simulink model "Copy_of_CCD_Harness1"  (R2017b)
settings: Solver=FixedStepDiscrete  StartTime=0.0  StopTime=10.0  FixedStep=0.01  RelTol=1e-3
undefined symbols (not defined in the file): sigbuilder_block

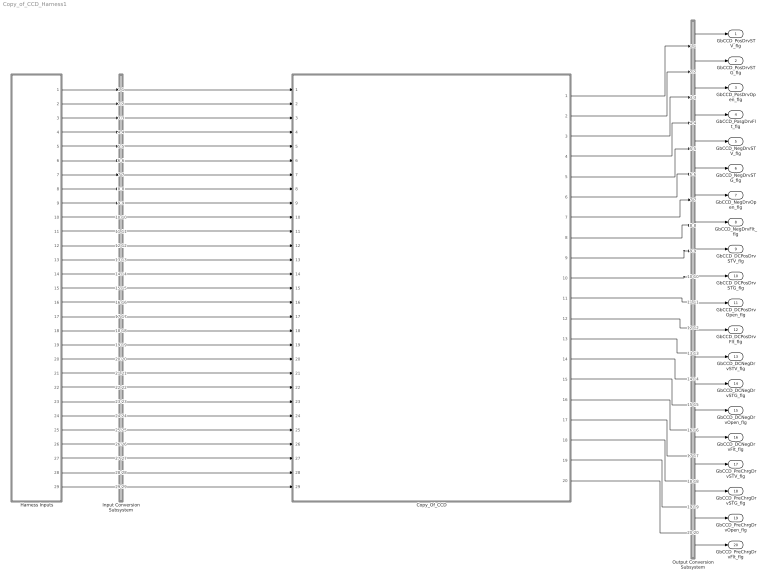
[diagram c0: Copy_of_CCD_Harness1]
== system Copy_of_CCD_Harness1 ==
  Copy_Of_CCD : ModelReference  ModelNameDialog=Copy_Of_CCD  SimulationMode=Normal  ModelReferenceVersion=1.11
  Harness Inputs : Subsystem  Tag=STV Subsys  LoadFcn=sigbuilder_block('load');  StartFcn=sigbuilder_block('start');  StopFcn=sigbuilder_block('stop');  ClipboardFcn=sigbuilder_block('clipboard');  mask(Sigbuilder block){tuvar=[0:10]}
      mask init:
      | if ~strcmp(get_param(bdroot(gcb),'SimulationStatus'),'stopped'),tuvar = sigbuilder_block('maskInit'); end
  Input Conversion Subsystem : Subsystem  Tag=__SLT_ICS__  Description=Signal spec. and routing
  Output Conversion Subsystem : Subsystem  Tag=__SLT_OCS__  Description=Signal spec. and routing
  GbCCD_PosDrvSTV_flg : Outport  OutDataTypeStr=boolean  PortDimensions=[1]
  GbCCD_PosDrvSTG_flg : Outport  Port=2  OutDataTypeStr=boolean  PortDimensions=[1]
  GbCCD_PosDrvOpen_flg : Outport  Port=3  OutDataTypeStr=boolean  PortDimensions=[1]
  GbCCD_PosgDrvFlt_flg : Outport  Port=4  OutDataTypeStr=boolean  PortDimensions=[1]
  GbCCD_NegDrvSTV_flg : Outport  Port=5  OutDataTypeStr=boolean  PortDimensions=[1]
  GbCCD_NegDrvSTG_flg : Outport  Port=6  OutDataTypeStr=boolean  PortDimensions=[1]
  GbCCD_NegDrvOpen_flg : Outport  Port=7  OutDataTypeStr=boolean  PortDimensions=[1]
  GbCCD_NegDrvFlt_flg : Outport  Port=8  OutDataTypeStr=boolean  PortDimensions=[1]
  GbCCD_DCPosDrvSTV_flg : Outport  Port=9  OutDataTypeStr=boolean  PortDimensions=[1]
  GbCCD_DCPosDrvSTG_flg : Outport  Port=10  OutDataTypeStr=boolean  PortDimensions=[1]
  GbCCD_DCPosDrvOpen_flg : Outport  Port=11  OutDataTypeStr=boolean  PortDimensions=[1]
  GbCCD_DCPosDrvFlt_flg : Outport  Port=12  OutDataTypeStr=boolean  PortDimensions=[1]
  GbCCD_DCNegDrvSTV_flg : Outport  Port=13  OutDataTypeStr=boolean  PortDimensions=[1]
  GbCCD_DCNegDrvSTG_flg : Outport  Port=14  OutDataTypeStr=boolean  PortDimensions=[1]
  GbCCD_DCNegDrvOpen_flg : Outport  Port=15  OutDataTypeStr=boolean  PortDimensions=[1]
  GbCCD_DCNegDrvFlt_flg : Outport  Port=16  OutDataTypeStr=boolean  PortDimensions=[1]
  GbCCD_PreChrgDrvSTV_flg : Outport  Port=17  OutDataTypeStr=boolean  PortDimensions=[1]
  GbCCD_PreChrgDrvSTG_flg : Outport  Port=18  OutDataTypeStr=boolean  PortDimensions=[1]
  GbCCD_PreChrgDrvOpen_flg : Outport  Port=19  OutDataTypeStr=boolean  PortDimensions=[1]
  GbCCD_PreChrgDrvFlt_flg : Outport  Port=20  OutDataTypeStr=boolean  PortDimensions=[1]
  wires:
  Harness Inputs/1(GcLDP_PosHsdCrnt_mV) -> Input Conversion Subsystem/1(Inport_1)
  Harness Inputs/2(GcLDP_ChrgPosHsdCrnt_mV) -> Input Conversion Subsystem/2(Inport_2)
  Harness Inputs/3(GcLDP_NegHsdCrnt_mV) -> Input Conversion Subsystem/3(Inport_3)
  Harness Inputs/4(GcLDP_ChrgPosHsdVolt_mV) -> Input Conversion Subsystem/4(Inport_4)
  Harness Inputs/5(GcLDP_ChrgNegHsdVolt_mV) -> Input Conversion Subsystem/5(Inport_5)
  Harness Inputs/6(GcLDP_PosHsdVolt_mV) -> Input Conversion Subsystem/6(Inport_6)
  Harness Inputs/7(GcLDP_NegHsdVolt_mV) -> Input Conversion Subsystem/7(Inport_7)
  Harness Inputs/8(GcISP_ChrgPosLsdDiag_numb) -> Input Conversion Subsystem/8(Inport_8)
  Harness Inputs/9(GcISP_ChrgNegLsdDiag_numb) -> Input Conversion Subsystem/9(Inport_9)
  Harness Inputs/10(GcISP_PosLsdDiag_numb) -> Input Conversion Subsystem/10(Inport_10)
  Harness Inputs/11(GcISP_NegLsdDiag_numb) -> Input Conversion Subsystem/11(Inport_11)
  Harness Inputs/12(GbCTC_PosCtlState_flg) -> Input Conversion Subsystem/12(Inport_12)
  Harness Inputs/13(GbCTC_NegCtlState_flg) -> Input Conversion Subsystem/13(Inport_13)
  Harness Inputs/14(GbCTC_DCPosChrgCtlState_flg) -> Input Conversion Subsystem/14(Inport_14)
  Harness Inputs/15(GbCTC_DCNegChrgCtlState_flg) -> Input Conversion Subsystem/15(Inport_15)
  Harness Inputs/16(GbLDP_PosHsdCrntVld_flg) -> Input Conversion Subsystem/16(Inport_16)
  Harness Inputs/17(GbLDP_ChrgPosHsdCrntVld_flg) -> Input Conversion Subsystem/17(Inport_17)
  Harness Inputs/18(GbLDP_NegHsdCrntVld_flg) -> Input Conversion Subsystem/18(Inport_18)
  Harness Inputs/19(GbLDP_ChrgNegHsdCrntVld_flg) -> Input Conversion Subsystem/19(Inport_19)
  Harness Inputs/20(GbLDP_ChrgPosHsdVoltVld_flg) -> Input Conversion Subsystem/20(Inport_20)
  Harness Inputs/21(GbLDP_ChrgNegHsdVoltVld_flg) -> Input Conversion Subsystem/21(Inport_21)
  Harness Inputs/22(GbLDP_PosHsdVoltVld_flg) -> Input Conversion Subsystem/22(Inport_22)
  Harness Inputs/23(GbLDP_NegHsdVoltVld_flg) -> Input Conversion Subsystem/23(Inport_23)
  Harness Inputs/24(GcLDP_Kl30Volt_mV) -> Input Conversion Subsystem/24(Inport_24)
  Harness Inputs/25(GcLDP_ChrgNegHsdCrnt_mV) -> Input Conversion Subsystem/25(Inport_25)
  Harness Inputs/26(GeUDS_AreaSel_enum) -> Input Conversion Subsystem/26(Inport_26)
  Harness Inputs/27(GcISP_PreLsdDiag_numb) -> Input Conversion Subsystem/27(Inport_27)
  Harness Inputs/28(GbCTC_PreChrgCtlState_flg) -> Input Conversion Subsystem/28(Inport_28)
  Harness Inputs/29(GcLDP_Kl30CVolt_mV1) -> Input Conversion Subsystem/29(Inport_29)
  Output Conversion Subsystem/1(Outport_1) -> GbCCD_PosDrvSTV_flg/1
  Output Conversion Subsystem/2(Outport_2) -> GbCCD_PosDrvSTG_flg/1
  Output Conversion Subsystem/3(Outport_3) -> GbCCD_PosDrvOpen_flg/1
  Output Conversion Subsystem/4(Outport_4) -> GbCCD_PosgDrvFlt_flg/1
  Output Conversion Subsystem/5(Outport_5) -> GbCCD_NegDrvSTV_flg/1
  Output Conversion Subsystem/6(Outport_6) -> GbCCD_NegDrvSTG_flg/1
  Output Conversion Subsystem/7(Outport_7) -> GbCCD_NegDrvOpen_flg/1
  Output Conversion Subsystem/8(Outport_8) -> GbCCD_NegDrvFlt_flg/1
  Output Conversion Subsystem/9(Outport_9) -> GbCCD_DCPosDrvSTV_flg/1
  Output Conversion Subsystem/10(Outport_10) -> GbCCD_DCPosDrvSTG_flg/1
  Output Conversion Subsystem/11(Outport_11) -> GbCCD_DCPosDrvOpen_flg/1
  Output Conversion Subsystem/12(Outport_12) -> GbCCD_DCPosDrvFlt_flg/1
  Output Conversion Subsystem/13(Outport_13) -> GbCCD_DCNegDrvSTV_flg/1
  Output Conversion Subsystem/14(Outport_14) -> GbCCD_DCNegDrvSTG_flg/1
  Output Conversion Subsystem/15(Outport_15) -> GbCCD_DCNegDrvOpen_flg/1
  Output Conversion Subsystem/16(Outport_16) -> GbCCD_DCNegDrvFlt_flg/1
  Output Conversion Subsystem/17(Outport_17) -> GbCCD_PreChrgDrvSTV_flg/1
  Output Conversion Subsystem/18(Outport_18) -> GbCCD_PreChrgDrvSTG_flg/1
  Output Conversion Subsystem/19(Outport_19) -> GbCCD_PreChrgDrvOpen_flg/1
  Output Conversion Subsystem/20(Outport_20) -> GbCCD_PreChrgDrvFlt_flg/1
  Input Conversion Subsystem/1(Outport_1) -> Copy_Of_CCD/1
  Input Conversion Subsystem/2(Outport_2) -> Copy_Of_CCD/2
  Input Conversion Subsystem/3(Outport_3) -> Copy_Of_CCD/3
  Input Conversion Subsystem/4(Outport_4) -> Copy_Of_CCD/4
  Input Conversion Subsystem/5(Outport_5) -> Copy_Of_CCD/5
  Input Conversion Subsystem/6(Outport_6) -> Copy_Of_CCD/6
  Input Conversion Subsystem/7(Outport_7) -> Copy_Of_CCD/7
  Input Conversion Subsystem/8(Outport_8) -> Copy_Of_CCD/8
  Input Conversion Subsystem/9(Outport_9) -> Copy_Of_CCD/9
  Input Conversion Subsystem/10(Outport_10) -> Copy_Of_CCD/10
  Input Conversion Subsystem/11(Outport_11) -> Copy_Of_CCD/11
  Input Conversion Subsystem/12(Outport_12) -> Copy_Of_CCD/12
  Input Conversion Subsystem/13(Outport_13) -> Copy_Of_CCD/13
  Input Conversion Subsystem/14(Outport_14) -> Copy_Of_CCD/14
  Input Conversion Subsystem/15(Outport_15) -> Copy_Of_CCD/15
  Input Conversion Subsystem/16(Outport_16) -> Copy_Of_CCD/16
  Input Conversion Subsystem/17(Outport_17) -> Copy_Of_CCD/17
  Input Conversion Subsystem/18(Outport_18) -> Copy_Of_CCD/18
  Input Conversion Subsystem/19(Outport_19) -> Copy_Of_CCD/19
  Input Conversion Subsystem/20(Outport_20) -> Copy_Of_CCD/20
  Input Conversion Subsystem/21(Outport_21) -> Copy_Of_CCD/21
  Input Conversion Subsystem/22(Outport_22) -> Copy_Of_CCD/22
  Input Conversion Subsystem/23(Outport_23) -> Copy_Of_CCD/23
  Input Conversion Subsystem/24(Outport_24) -> Copy_Of_CCD/24
  Input Conversion Subsystem/25(Outport_25) -> Copy_Of_CCD/25
  Input Conversion Subsystem/26(Outport_26) -> Copy_Of_CCD/26
  Input Conversion Subsystem/27(Outport_27) -> Copy_Of_CCD/27
  Input Conversion Subsystem/28(Outport_28) -> Copy_Of_CCD/28
  Input Conversion Subsystem/29(Outport_29) -> Copy_Of_CCD/29
  Copy_Of_CCD/1 -> Output Conversion Subsystem/1(Inport_1)
  Copy_Of_CCD/2 -> Output Conversion Subsystem/2(Inport_2)
  Copy_Of_CCD/3 -> Output Conversion Subsystem/3(Inport_3)
  Copy_Of_CCD/4 -> Output Conversion Subsystem/4(Inport_4)
  Copy_Of_CCD/5 -> Output Conversion Subsystem/5(Inport_5)
  Copy_Of_CCD/6 -> Output Conversion Subsystem/6(Inport_6)
  Copy_Of_CCD/7 -> Output Conversion Subsystem/7(Inport_7)
  Copy_Of_CCD/8 -> Output Conversion Subsystem/8(Inport_8)
  Copy_Of_CCD/9 -> Output Conversion Subsystem/9(Inport_9)
  Copy_Of_CCD/10 -> Output Conversion Subsystem/10(Inport_10)
  Copy_Of_CCD/11 -> Output Conversion Subsystem/11(Inport_11)
  Copy_Of_CCD/12 -> Output Conversion Subsystem/12(Inport_12)
  Copy_Of_CCD/13 -> Output Conversion Subsystem/13(Inport_13)
  Copy_Of_CCD/14 -> Output Conversion Subsystem/14(Inport_14)
  Copy_Of_CCD/15 -> Output Conversion Subsystem/15(Inport_15)
  Copy_Of_CCD/16 -> Output Conversion Subsystem/16(Inport_16)
  Copy_Of_CCD/17 -> Output Conversion Subsystem/17(Inport_17)
  Copy_Of_CCD/18 -> Output Conversion Subsystem/18(Inport_18)
  Copy_Of_CCD/19 -> Output Conversion Subsystem/19(Inport_19)
  Copy_Of_CCD/20 -> Output Conversion Subsystem/20(Inport_20)

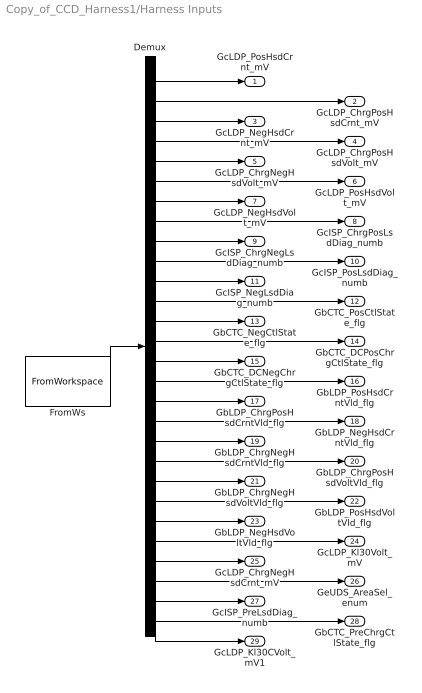
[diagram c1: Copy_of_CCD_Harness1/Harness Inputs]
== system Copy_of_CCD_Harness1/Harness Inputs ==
  Demux : Demux  Tag=STV Demux  Outputs=29
  FromWs : FromWorkspace  Tag=STV FromWs  VariableName=tuvar  SampleTime=0
  GcLDP_PosHsdCrnt_mV : Outport  Tag=STV Outport
  GcLDP_ChrgPosHsdCrnt_mV : Outport  Tag=STV Outport  Port=2
  GcLDP_NegHsdCrnt_mV : Outport  Tag=STV Outport  Port=3
  GcLDP_ChrgPosHsdVolt_mV : Outport  Tag=STV Outport  Port=4
  GcLDP_ChrgNegHsdVolt_mV : Outport  Tag=STV Outport  Port=5
  GcLDP_PosHsdVolt_mV : Outport  Tag=STV Outport  Port=6
  GcLDP_NegHsdVolt_mV : Outport  Tag=STV Outport  Port=7
  GcISP_ChrgPosLsdDiag_numb : Outport  Tag=STV Outport  Port=8
  GcISP_ChrgNegLsdDiag_numb : Outport  Tag=STV Outport  Port=9
  GcISP_PosLsdDiag_numb : Outport  Tag=STV Outport  Port=10
  GcISP_NegLsdDiag_numb : Outport  Tag=STV Outport  Port=11
  GbCTC_PosCtlState_flg : Outport  Tag=STV Outport  Port=12
  GbCTC_NegCtlState_flg : Outport  Tag=STV Outport  Port=13
  GbCTC_DCPosChrgCtlState_flg : Outport  Tag=STV Outport  Port=14
  GbCTC_DCNegChrgCtlState_flg : Outport  Tag=STV Outport  Port=15
  GbLDP_PosHsdCrntVld_flg : Outport  Tag=STV Outport  Port=16
  GbLDP_ChrgPosHsdCrntVld_flg : Outport  Tag=STV Outport  Port=17
  GbLDP_NegHsdCrntVld_flg : Outport  Tag=STV Outport  Port=18
  GbLDP_ChrgNegHsdCrntVld_flg : Outport  Tag=STV Outport  Port=19
  GbLDP_ChrgPosHsdVoltVld_flg : Outport  Tag=STV Outport  Port=20
  GbLDP_ChrgNegHsdVoltVld_flg : Outport  Tag=STV Outport  Port=21
  GbLDP_PosHsdVoltVld_flg : Outport  Tag=STV Outport  Port=22
  GbLDP_NegHsdVoltVld_flg : Outport  Tag=STV Outport  Port=23
  GcLDP_Kl30Volt_mV : Outport  Tag=STV Outport  Port=24
  GcLDP_ChrgNegHsdCrnt_mV : Outport  Tag=STV Outport  Port=25
  GeUDS_AreaSel_enum : Outport  Tag=STV Outport  Port=26
  GcISP_PreLsdDiag_numb : Outport  Tag=STV Outport  Port=27
  GbCTC_PreChrgCtlState_flg : Outport  Tag=STV Outport  Port=28
  GcLDP_Kl30CVolt_mV1 : Outport  Tag=STV Outport  Port=29
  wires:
  FromWs/1 -> Demux/1
  Demux/1 -> GcLDP_PosHsdCrnt_mV/1
  Demux/2 -> GcLDP_ChrgPosHsdCrnt_mV/1
  Demux/3 -> GcLDP_NegHsdCrnt_mV/1
  Demux/4 -> GcLDP_ChrgPosHsdVolt_mV/1
  Demux/5 -> GcLDP_ChrgNegHsdVolt_mV/1
  Demux/6 -> GcLDP_PosHsdVolt_mV/1
  Demux/7 -> GcLDP_NegHsdVolt_mV/1
  Demux/8 -> GcISP_ChrgPosLsdDiag_numb/1
  Demux/9 -> GcISP_ChrgNegLsdDiag_numb/1
  Demux/10 -> GcISP_PosLsdDiag_numb/1
  Demux/11 -> GcISP_NegLsdDiag_numb/1
  Demux/12 -> GbCTC_PosCtlState_flg/1
  Demux/13 -> GbCTC_NegCtlState_flg/1
  Demux/14 -> GbCTC_DCPosChrgCtlState_flg/1
  Demux/15 -> GbCTC_DCNegChrgCtlState_flg/1
  Demux/16 -> GbLDP_PosHsdCrntVld_flg/1
  Demux/17 -> GbLDP_ChrgPosHsdCrntVld_flg/1
  Demux/18 -> GbLDP_NegHsdCrntVld_flg/1
  Demux/19 -> GbLDP_ChrgNegHsdCrntVld_flg/1
  Demux/20 -> GbLDP_ChrgPosHsdVoltVld_flg/1
  Demux/21 -> GbLDP_ChrgNegHsdVoltVld_flg/1
  Demux/22 -> GbLDP_PosHsdVoltVld_flg/1
  Demux/23 -> GbLDP_NegHsdVoltVld_flg/1
  Demux/24 -> GcLDP_Kl30Volt_mV/1
  Demux/25 -> GcLDP_ChrgNegHsdCrnt_mV/1
  Demux/26 -> GeUDS_AreaSel_enum/1
  Demux/27 -> GcISP_PreLsdDiag_numb/1
  Demux/28 -> GbCTC_PreChrgCtlState_flg/1
  Demux/29 -> GcLDP_Kl30CVolt_mV1/1

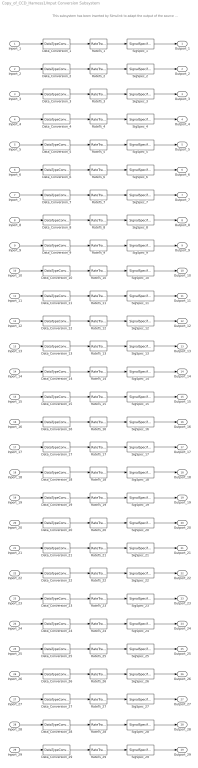
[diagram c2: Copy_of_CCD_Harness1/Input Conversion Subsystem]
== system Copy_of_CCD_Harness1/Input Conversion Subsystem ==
  note: This subsystem has been inserted by Simulink to adapt the output of the source blocks to the interface required by the harnessed component. Modifying the contents of this subsystem may result in compilation and simulation failure.
  Inport_1 : Inport
  Inport_2 : Inport  Port=2
  Inport_3 : Inport  Port=3
  Inport_4 : Inport  Port=4
  Inport_5 : Inport  Port=5
  Inport_6 : Inport  Port=6
  Inport_7 : Inport  Port=7
  Inport_8 : Inport  Port=8
  Inport_9 : Inport  Port=9
  Inport_10 : Inport  Port=10
  Inport_11 : Inport  Port=11
  Inport_12 : Inport  Port=12
  Inport_13 : Inport  Port=13
  Inport_14 : Inport  Port=14
  Inport_15 : Inport  Port=15
  Inport_16 : Inport  Port=16
  Inport_17 : Inport  Port=17
  Inport_18 : Inport  Port=18
  Inport_19 : Inport  Port=19
  Inport_20 : Inport  Port=20
  Inport_21 : Inport  Port=21
  Inport_22 : Inport  Port=22
  Inport_23 : Inport  Port=23
  Inport_24 : Inport  Port=24
  Inport_25 : Inport  Port=25
  Inport_26 : Inport  Port=26
  Inport_27 : Inport  Port=27
  Inport_28 : Inport  Port=28
  Inport_29 : Inport  Port=29
  Data_Conversion_{1..7,24..25,29} (10 alike) : DataTypeConversion  OutDataTypeStr=uint16
  Data_Conversion_{8..11,26..27} (6 alike) : DataTypeConversion  OutDataTypeStr=uint8
  Data_Conversion_{12..23,28} (13 alike) : DataTypeConversion  OutDataTypeStr=boolean
  RateTs_{1..29} (29 alike) : RateTransition  OutPortSampleTime=0.01
  SigSpec_{1..7,24..25,29} (10 alike) : SignalSpecification  OutDataTypeStr=uint16  Unit=mv  Dimensions=[1]  SampleTime=0.01
  SigSpec_{8..11,27} (5 alike) : SignalSpecification  OutDataTypeStr=uint8  Unit=numb  Dimensions=[1]  SampleTime=0.01
  SigSpec_{12..23,28} (13 alike) : SignalSpecification  OutDataTypeStr=boolean  Unit=flg  Dimensions=[1]  SampleTime=0.01
  SigSpec_26 : SignalSpecification  OutDataTypeStr=uint8  Unit=enum  Dimensions=[1]  SampleTime=0.01
  Outport_1 : Outport
  Outport_2 : Outport  Port=2
  Outport_3 : Outport  Port=3
  Outport_4 : Outport  Port=4
  Outport_5 : Outport  Port=5
  Outport_6 : Outport  Port=6
  Outport_7 : Outport  Port=7
  Outport_8 : Outport  Port=8
  Outport_9 : Outport  Port=9
  Outport_10 : Outport  Port=10
  Outport_11 : Outport  Port=11
  Outport_12 : Outport  Port=12
  Outport_13 : Outport  Port=13
  Outport_14 : Outport  Port=14
  Outport_15 : Outport  Port=15
  Outport_16 : Outport  Port=16
  Outport_17 : Outport  Port=17
  Outport_18 : Outport  Port=18
  Outport_19 : Outport  Port=19
  Outport_20 : Outport  Port=20
  Outport_21 : Outport  Port=21
  Outport_22 : Outport  Port=22
  Outport_23 : Outport  Port=23
  Outport_24 : Outport  Port=24
  Outport_25 : Outport  Port=25
  Outport_26 : Outport  Port=26
  Outport_27 : Outport  Port=27
  Outport_28 : Outport  Port=28
  Outport_29 : Outport  Port=29
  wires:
  SigSpec_1/1 -> Outport_1/1
  RateTs_1/1 -> SigSpec_1/1
  Data_Conversion_1/1 -> RateTs_1/1
  Inport_1/1 -> Data_Conversion_1/1
  SigSpec_2/1 -> Outport_2/1
  RateTs_2/1 -> SigSpec_2/1
  Data_Conversion_2/1 -> RateTs_2/1
  Inport_2/1 -> Data_Conversion_2/1
  SigSpec_3/1 -> Outport_3/1
  RateTs_3/1 -> SigSpec_3/1
  Data_Conversion_3/1 -> RateTs_3/1
  Inport_3/1 -> Data_Conversion_3/1
  SigSpec_4/1 -> Outport_4/1
  RateTs_4/1 -> SigSpec_4/1
  Data_Conversion_4/1 -> RateTs_4/1
  Inport_4/1 -> Data_Conversion_4/1
  SigSpec_5/1 -> Outport_5/1
  RateTs_5/1 -> SigSpec_5/1
  Data_Conversion_5/1 -> RateTs_5/1
  Inport_5/1 -> Data_Conversion_5/1
  SigSpec_6/1 -> Outport_6/1
  RateTs_6/1 -> SigSpec_6/1
  Data_Conversion_6/1 -> RateTs_6/1
  Inport_6/1 -> Data_Conversion_6/1
  SigSpec_7/1 -> Outport_7/1
  RateTs_7/1 -> SigSpec_7/1
  Data_Conversion_7/1 -> RateTs_7/1
  Inport_7/1 -> Data_Conversion_7/1
  SigSpec_8/1 -> Outport_8/1
  RateTs_8/1 -> SigSpec_8/1
  Data_Conversion_8/1 -> RateTs_8/1
  Inport_8/1 -> Data_Conversion_8/1
  SigSpec_9/1 -> Outport_9/1
  RateTs_9/1 -> SigSpec_9/1
  Data_Conversion_9/1 -> RateTs_9/1
  Inport_9/1 -> Data_Conversion_9/1
  SigSpec_10/1 -> Outport_10/1
  RateTs_10/1 -> SigSpec_10/1
  Data_Conversion_10/1 -> RateTs_10/1
  Inport_10/1 -> Data_Conversion_10/1
  SigSpec_11/1 -> Outport_11/1
  RateTs_11/1 -> SigSpec_11/1
  Data_Conversion_11/1 -> RateTs_11/1
  Inport_11/1 -> Data_Conversion_11/1
  SigSpec_12/1 -> Outport_12/1
  RateTs_12/1 -> SigSpec_12/1
  Data_Conversion_12/1 -> RateTs_12/1
  Inport_12/1 -> Data_Conversion_12/1
  SigSpec_13/1 -> Outport_13/1
  RateTs_13/1 -> SigSpec_13/1
  Data_Conversion_13/1 -> RateTs_13/1
  Inport_13/1 -> Data_Conversion_13/1
  SigSpec_14/1 -> Outport_14/1
  RateTs_14/1 -> SigSpec_14/1
  Data_Conversion_14/1 -> RateTs_14/1
  Inport_14/1 -> Data_Conversion_14/1
  SigSpec_15/1 -> Outport_15/1
  RateTs_15/1 -> SigSpec_15/1
  Data_Conversion_15/1 -> RateTs_15/1
  Inport_15/1 -> Data_Conversion_15/1
  SigSpec_16/1 -> Outport_16/1
  RateTs_16/1 -> SigSpec_16/1
  Data_Conversion_16/1 -> RateTs_16/1
  Inport_16/1 -> Data_Conversion_16/1
  SigSpec_17/1 -> Outport_17/1
  RateTs_17/1 -> SigSpec_17/1
  Data_Conversion_17/1 -> RateTs_17/1
  Inport_17/1 -> Data_Conversion_17/1
  SigSpec_18/1 -> Outport_18/1
  RateTs_18/1 -> SigSpec_18/1
  Data_Conversion_18/1 -> RateTs_18/1
  Inport_18/1 -> Data_Conversion_18/1
  SigSpec_19/1 -> Outport_19/1
  RateTs_19/1 -> SigSpec_19/1
  Data_Conversion_19/1 -> RateTs_19/1
  Inport_19/1 -> Data_Conversion_19/1
  SigSpec_20/1 -> Outport_20/1
  RateTs_20/1 -> SigSpec_20/1
  Data_Conversion_20/1 -> RateTs_20/1
  Inport_20/1 -> Data_Conversion_20/1
  SigSpec_21/1 -> Outport_21/1
  RateTs_21/1 -> SigSpec_21/1
  Data_Conversion_21/1 -> RateTs_21/1
  Inport_21/1 -> Data_Conversion_21/1
  SigSpec_22/1 -> Outport_22/1
  RateTs_22/1 -> SigSpec_22/1
  Data_Conversion_22/1 -> RateTs_22/1
  Inport_22/1 -> Data_Conversion_22/1
  SigSpec_23/1 -> Outport_23/1
  RateTs_23/1 -> SigSpec_23/1
  Data_Conversion_23/1 -> RateTs_23/1
  Inport_23/1 -> Data_Conversion_23/1
  SigSpec_24/1 -> Outport_24/1
  RateTs_24/1 -> SigSpec_24/1
  Data_Conversion_24/1 -> RateTs_24/1
  Inport_24/1 -> Data_Conversion_24/1
  SigSpec_25/1 -> Outport_25/1
  RateTs_25/1 -> SigSpec_25/1
  Data_Conversion_25/1 -> RateTs_25/1
  Inport_25/1 -> Data_Conversion_25/1
  SigSpec_26/1 -> Outport_26/1
  RateTs_26/1 -> SigSpec_26/1
  Data_Conversion_26/1 -> RateTs_26/1
  Inport_26/1 -> Data_Conversion_26/1
  SigSpec_27/1 -> Outport_27/1
  RateTs_27/1 -> SigSpec_27/1
  Data_Conversion_27/1 -> RateTs_27/1
  Inport_27/1 -> Data_Conversion_27/1
  SigSpec_28/1 -> Outport_28/1
  RateTs_28/1 -> SigSpec_28/1
  Data_Conversion_28/1 -> RateTs_28/1
  Inport_28/1 -> Data_Conversion_28/1
  SigSpec_29/1 -> Outport_29/1
  RateTs_29/1 -> SigSpec_29/1
  Data_Conversion_29/1 -> RateTs_29/1
  Inport_29/1 -> Data_Conversion_29/1

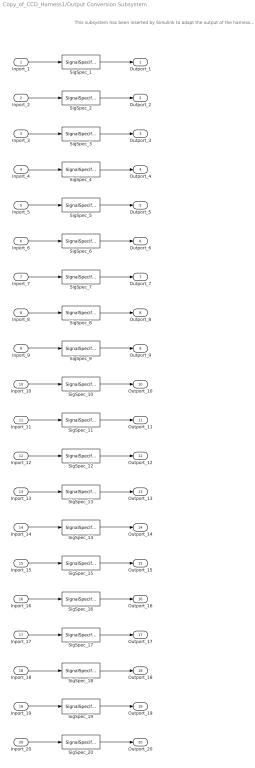
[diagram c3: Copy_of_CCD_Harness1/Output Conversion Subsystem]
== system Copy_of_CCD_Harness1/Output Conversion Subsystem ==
  note: This subsystem has been inserted by Simulink to adapt the output of the harnessed component to the interface required by the sink blocks. Modifying the contents of this subsystem may result in compilation and simulation failure.
  Inport_1 : Inport
  Inport_2 : Inport  Port=2
  Inport_3 : Inport  Port=3
  Inport_4 : Inport  Port=4
  Inport_5 : Inport  Port=5
  Inport_6 : Inport  Port=6
  Inport_7 : Inport  Port=7
  Inport_8 : Inport  Port=8
  Inport_9 : Inport  Port=9
  Inport_10 : Inport  Port=10
  Inport_11 : Inport  Port=11
  Inport_12 : Inport  Port=12
  Inport_13 : Inport  Port=13
  Inport_14 : Inport  Port=14
  Inport_15 : Inport  Port=15
  Inport_16 : Inport  Port=16
  Inport_17 : Inport  Port=17
  Inport_18 : Inport  Port=18
  Inport_19 : Inport  Port=19
  Inport_20 : Inport  Port=20
  SigSpec_{1..20} (20 alike) : SignalSpecification  OutDataTypeStr=boolean  Unit=flag  Dimensions=[1]  SampleTime=0.01
  Outport_1 : Outport
  Outport_2 : Outport  Port=2
  Outport_3 : Outport  Port=3
  Outport_4 : Outport  Port=4
  Outport_5 : Outport  Port=5
  Outport_6 : Outport  Port=6
  Outport_7 : Outport  Port=7
  Outport_8 : Outport  Port=8
  Outport_9 : Outport  Port=9
  Outport_10 : Outport  Port=10
  Outport_11 : Outport  Port=11
  Outport_12 : Outport  Port=12
  Outport_13 : Outport  Port=13
  Outport_14 : Outport  Port=14
  Outport_15 : Outport  Port=15
  Outport_16 : Outport  Port=16
  Outport_17 : Outport  Port=17
  Outport_18 : Outport  Port=18
  Outport_19 : Outport  Port=19
  Outport_20 : Outport  Port=20
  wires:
  Inport_1/1 -> SigSpec_1/1
  SigSpec_1/1 -> Outport_1/1
  Inport_2/1 -> SigSpec_2/1
  SigSpec_2/1 -> Outport_2/1
  Inport_3/1 -> SigSpec_3/1
  SigSpec_3/1 -> Outport_3/1
  Inport_4/1 -> SigSpec_4/1
  SigSpec_4/1 -> Outport_4/1
  Inport_5/1 -> SigSpec_5/1
  SigSpec_5/1 -> Outport_5/1
  Inport_6/1 -> SigSpec_6/1
  SigSpec_6/1 -> Outport_6/1
  Inport_7/1 -> SigSpec_7/1
  SigSpec_7/1 -> Outport_7/1
  Inport_8/1 -> SigSpec_8/1
  SigSpec_8/1 -> Outport_8/1
  Inport_9/1 -> SigSpec_9/1
  SigSpec_9/1 -> Outport_9/1
  Inport_10/1 -> SigSpec_10/1
  SigSpec_10/1 -> Outport_10/1
  Inport_11/1 -> SigSpec_11/1
  SigSpec_11/1 -> Outport_11/1
  Inport_12/1 -> SigSpec_12/1
  SigSpec_12/1 -> Outport_12/1
  Inport_13/1 -> SigSpec_13/1
  SigSpec_13/1 -> Outport_13/1
  Inport_14/1 -> SigSpec_14/1
  SigSpec_14/1 -> Outport_14/1
  Inport_15/1 -> SigSpec_15/1
  SigSpec_15/1 -> Outport_15/1
  Inport_16/1 -> SigSpec_16/1
  SigSpec_16/1 -> Outport_16/1
  Inport_17/1 -> SigSpec_17/1
  SigSpec_17/1 -> Outport_17/1
  Inport_18/1 -> SigSpec_18/1
  SigSpec_18/1 -> Outport_18/1
  Inport_19/1 -> SigSpec_19/1
  SigSpec_19/1 -> Outport_19/1
  Inport_20/1 -> SigSpec_20/1
  SigSpec_20/1 -> Outport_20/1
